PROGRAM MAIN
VAR
	// Instance
	Ax1				:AXIS_REF;
	mcPower			:MC_Power;
	mcMovAbs		:MC_MoveAbsolute;
	mcMovVelo		:MC_MoveVelocity;
	mcJOG			:MC_Jog;
	mcReset			:MC_Reset;

	// App1
	bStartApp1			:BOOL;
	fbTrig_StartApp1	:R_TRIG;
	iStepApp1			:INT;
	bPauseApp1			:BOOL;
	fbTrig_PauseApp1	:R_TRIG;
	fbTrig_RestoreApp1	:F_TRIG;	
	bApp1Busy,
	bApp1Done,
	bApp1Error			:BOOL;
	
	// App2
	bStartApp2			:BOOL;
	bGoToNextStep		:BOOL;
	fbTrig_StartApp2	:R_TRIG;
	iStepApp2			:INT;
	bApp2Busy,
	bApp2Done,
	bApp2Error			:BOOL;	
	
	// App3
	bStartApp3			:BOOL;
	fbTrig_StartApp3	:R_TRIG;
	iStepApp3			:INT;
	lrManualOverride	:LREAL;
	bApp3Busy,
	bApp3Done,
	bApp3Error			:BOOL;	
END_VAR

// 轴实例调用
ACT_AxesInstance();

// 应用1：多段位移运动不打断流程暂停
bStartApp1;		bPauseApp1;// 控制信号
iStepApp1;	bApp1Busy;bApp1Done;bApp1Error;// 状态监控信号
ACT_App1();

// 应用2：Override=0时触发，满足条件后设为100执行动作
bStartApp2; 	bGoToNextStep;// 控制信号
iStepApp2;	bApp2Busy;bApp2Done;bApp2Error;// 状态监控信号
ACT_App2();

// 应用3：Visu手动控制，无级变速
ACT_App3();

ACTION ACT_App1:
(*
	动作描述：
		—>启动
		—>TargetPos=0
		—>TargetPos=100
		—>TargetPos=200
		—>TargetPos=300
		—>TargetPos=400
		—>TargetPos=500
		—>TargetPos=0
		—>结束
*)
fbTrig_PauseApp1(CLK:=bPauseApp1);
fbTrig_RestoreApp1(CLK:=bPauseApp1);
IF fbTrig_PauseApp1.Q THEN
	mcPower.Override := 0;
ELSIF fbTrig_RestoreApp1.Q THEN
	mcPower.Override := 100;
END_IF


fbTrig_StartApp1(CLK:=bStartApp1);
IF fbTrig_StartApp1.Q 
	AND NOT bApp1Busy THEN
	iStepApp1 := 10;
END_IF

CASE iStepApp1 OF
	0:
		;
		
	10:
		mcPower.Override := 100;
		mcReset(Axis:=Ax1,Execute:=FALSE);
		mcReset(Axis:=Ax1,Execute:=TRUE);
		iStepApp1 := iStepApp1 + 10;
		
	20:
		IF NOT mcReset.Busy THEN
			IF mcReset.Done THEN
				iStepApp1 := iStepApp1 + 10;
			ELSE
				iStepApp1 := 999;
			END_IF
			mcReset(Axis:=Ax1,Execute:=FALSE);
		END_IF
		
	// Target = 0	
	30:
		mcMovAbs.Position := 0;
		mcMovAbs.Velocity := 50;
		mcMovAbs(Axis:=Ax1,Execute:=FALSE);
		mcMovAbs(Axis:=Ax1,Execute:=TRUE);
		iStepApp1 := iStepApp1 + 10;
		
	40:
		IF NOT mcMovAbs.Busy THEN
			IF mcMovAbs.Done THEN
				iStepApp1 := iStepApp1 + 10;
			ELSE
				iStepApp1 := 999;
			END_IF
			mcMovAbs(Axis:=Ax1,Execute:=FALSE);
		END_IF
		
	// Target = 100	
	50:
		mcMovAbs.Position := 100;
		mcMovAbs.Velocity := 50;
		mcMovAbs(Axis:=Ax1,Execute:=FALSE);
		mcMovAbs(Axis:=Ax1,Execute:=TRUE);
		iStepApp1 := iStepApp1 + 10;
		
	60:
		IF NOT mcMovAbs.Busy THEN
			IF mcMovAbs.Done THEN
				iStepApp1 := iStepApp1 + 10;
			ELSE
				iStepApp1 := 999;
			END_IF
			mcMovAbs(Axis:=Ax1,Execute:=FALSE);
		END_IF	
		
	// Target = 200	
	70:
		mcMovAbs.Position := 200;
		mcMovAbs.Velocity := 50;
		mcMovAbs(Axis:=Ax1,Execute:=FALSE);
		mcMovAbs(Axis:=Ax1,Execute:=TRUE);
		iStepApp1 := iStepApp1 + 10;
		
	80:
		IF NOT mcMovAbs.Busy THEN
			IF mcMovAbs.Done THEN
				iStepApp1 := iStepApp1 + 10;
			ELSE
				iStepApp1 := 999;
			END_IF
			mcMovAbs(Axis:=Ax1,Execute:=FALSE);
		END_IF	
	
	// Target = 300	
	90:
		mcMovAbs.Position := 300;
		mcMovAbs.Velocity := 50;
		mcMovAbs(Axis:=Ax1,Execute:=FALSE);
		mcMovAbs(Axis:=Ax1,Execute:=TRUE);
		iStepApp1 := iStepApp1 + 10;
		
	100:
		IF NOT mcMovAbs.Busy THEN
			IF mcMovAbs.Done THEN
				iStepApp1 := iStepApp1 + 10;
			ELSE
				iStepApp1 := 999;
			END_IF
			mcMovAbs(Axis:=Ax1,Execute:=FALSE);
		END_IF

	// Target = 400	
	110:
		mcMovAbs.Position := 400;
		mcMovAbs.Velocity := 50;
		mcMovAbs(Axis:=Ax1,Execute:=FALSE);
		mcMovAbs(Axis:=Ax1,Execute:=TRUE);
		iStepApp1 := iStepApp1 + 10;
		
	120:
		IF NOT mcMovAbs.Busy THEN
			IF mcMovAbs.Done THEN
				iStepApp1 := iStepApp1 + 10;
			ELSE
				iStepApp1 := 999;
			END_IF
			mcMovAbs(Axis:=Ax1,Execute:=FALSE);
		END_IF

	// Target = 500	
	130:
		mcMovAbs.Position := 500;
		mcMovAbs.Velocity := 50;
		mcMovAbs(Axis:=Ax1,Execute:=FALSE);
		mcMovAbs(Axis:=Ax1,Execute:=TRUE);
		iStepApp1 := iStepApp1 + 10;
		
	140:
		IF NOT mcMovAbs.Busy THEN
			IF mcMovAbs.Done THEN
				iStepApp1 := iStepApp1 + 10;
			ELSE
				iStepApp1 := 999;
			END_IF
			mcMovAbs(Axis:=Ax1,Execute:=FALSE);
		END_IF	
		
	// Target = 0	
	150:
		mcMovAbs.Position := 0;
		mcMovAbs.Velocity := 50;
		mcMovAbs(Axis:=Ax1,Execute:=FALSE);
		mcMovAbs(Axis:=Ax1,Execute:=TRUE);
		iStepApp1 := iStepApp1 + 10;
		
	160:
		IF NOT mcMovAbs.Busy THEN
			IF mcMovAbs.Done THEN
				iStepApp1 := iStepApp1 + 10;
			ELSE
				iStepApp1 := 999;
			END_IF
			mcMovAbs(Axis:=Ax1,Execute:=FALSE);
		END_IF

	170,999:
		IF NOT bStartApp1 THEN
			iStepApp1 := 0;
		END_IF		
END_CASE
bApp1Busy := iStepApp1 >= 10 AND iStepApp1 <= 160;
bApp1Done := iStepApp1 = 170;
bApp1Error := iStepApp1 = 999;
END_ACTION

ACTION ACT_App2:
IF bGoToNextStep THEN
	bGoToNextStep := FALSE;
	mcPower.Override := 100;
END_IF

fbTrig_StartApp2(CLK:=bStartApp2);
IF fbTrig_StartApp2.Q
	AND NOT bApp2Busy THEN
	iStepApp2 := 10;
END_IF

CASE iStepApp2 OF
	0:
		;
		
	10:
		mcPower.Override := 0;
		mcReset(Axis:=Ax1,Execute:=FALSE);
		mcReset(Axis:=Ax1,Execute:=TRUE);
		iStepApp2 := iStepApp2 + 10;
		
	20:
		mcMovAbs.Position := 100;
		mcMovAbs.Velocity := 20;
		mcMovAbs(Axis:=Ax1, Execute := FALSE);
		mcMovAbs(Axis:=Ax1, Execute := TRUE);
		iStepApp2 := iStepApp2 + 10;
		
	30:
		IF NOT mcMovAbs.Busy THEN
			IF mcMovAbs.Done THEN
				iStepApp2 := iStepApp2 + 10;
			ELSE
				iStepApp2 := 999;
			END_IF
			mcMovAbs(Axis:=Ax1, Execute := FALSE);
		END_IF
		
	40,999:
		IF NOT bStartApp2 THEN
			iStepApp2 := 0;
		END_IF
END_CASE
bApp2Busy := iStepApp2 >= 10 AND iStepApp2 < 40;
bApp2Done := iStepApp2 = 40;
bApp2Error := iStepApp2 = 999;
END_ACTION

ACTION ACT_App3:
fbTrig_StartApp3(CLK := bStartApp3);
IF fbTrig_StartApp3.Q
	AND NOT bApp3Busy THEN
	iStepApp3 := 10;
END_IF

CASE iStepApp3 OF
	0:
		;
		
	10:
		mcPower.Override := 0;
		lrManualOverride := 0;
		mcReset(Axis:=Ax1,Execute:=FALSE);
		mcReset(Axis:=Ax1,Execute:=TRUE);
		iStepApp3 := iStepApp3 + 10;
		
	20:
		mcJOG.Velocity := 123;
		mcJOG(Axis:=Ax1, JogForward := FALSE, JogBackwards := FALSE);
		mcJOG(Axis:=Ax1, JogForward := TRUE, JogBackwards := FALSE);
		iStepApp3 := iStepApp3 + 10;
		
	30,999:
		mcPower.Override := lrManualOverride;
		IF NOT bStartApp3 THEN
			mcPower.Override := 0;
			lrManualOverride := 0;
			mcJOG(Axis:=Ax1, JogForward := FALSE, JogBackwards := FALSE);
			iStepApp3 := 0;
		END_IF		
END_CASE
END_ACTION

ACTION ACT_AxesInstance:
mcPower(
    Axis             := Ax1,
    Enable           := 1,
    Enable_Positive  := 1,
    Enable_Negative  := 1,
    Override         := ,
    BufferMode       := ,
    Options          := ,
    Status           => ,
    Busy             => ,
    Active           => ,
    Error            => ,
    ErrorID          => );
	
	
mcMovVelo(
    Axis            := Ax1,
    Execute         := ,
    Velocity        := ,
    Acceleration    := ,
    Deceleration    := ,
    Jerk            := ,
    Direction       := ,
    BufferMode      := ,
    Options         := ,
    InVelocity      => ,
    Busy            => ,
    Active          => ,
    CommandAborted  => ,
    Error           => ,
    ErrorID         => );
	
mcMovAbs(
    Axis            := Ax1,
    Execute         := ,
    Position        := ,
    Velocity        := ,
    Acceleration    := ,
    Deceleration    := ,
    Jerk            := ,
    BufferMode      := ,
    Options         := ,
    Done            => ,
    Busy            => ,
    Active          => ,
    CommandAborted  => ,
    Error           => ,
    ErrorID         => );

mcJOG(
    Axis            := Ax1,
    JogForward      := ,
    JogBackwards    := ,
    Mode            := E_JogMode.MC_JOGMODE_CONTINOUS,
    Position        := ,
    Velocity        := ,
    Acceleration    := ,
    Deceleration    := ,
    Jerk            := ,
    Done            => ,
    Busy            => ,
    Active          => ,
    CommandAborted  => ,
    Error           => ,
    ErrorID         => );
	
mcReset(
    Axis     := Ax1,
    Execute  := ,
    Done     => ,
    Busy     => ,
    Error    => ,
    ErrorID  => );
END_ACTION

END_PROGRAM
